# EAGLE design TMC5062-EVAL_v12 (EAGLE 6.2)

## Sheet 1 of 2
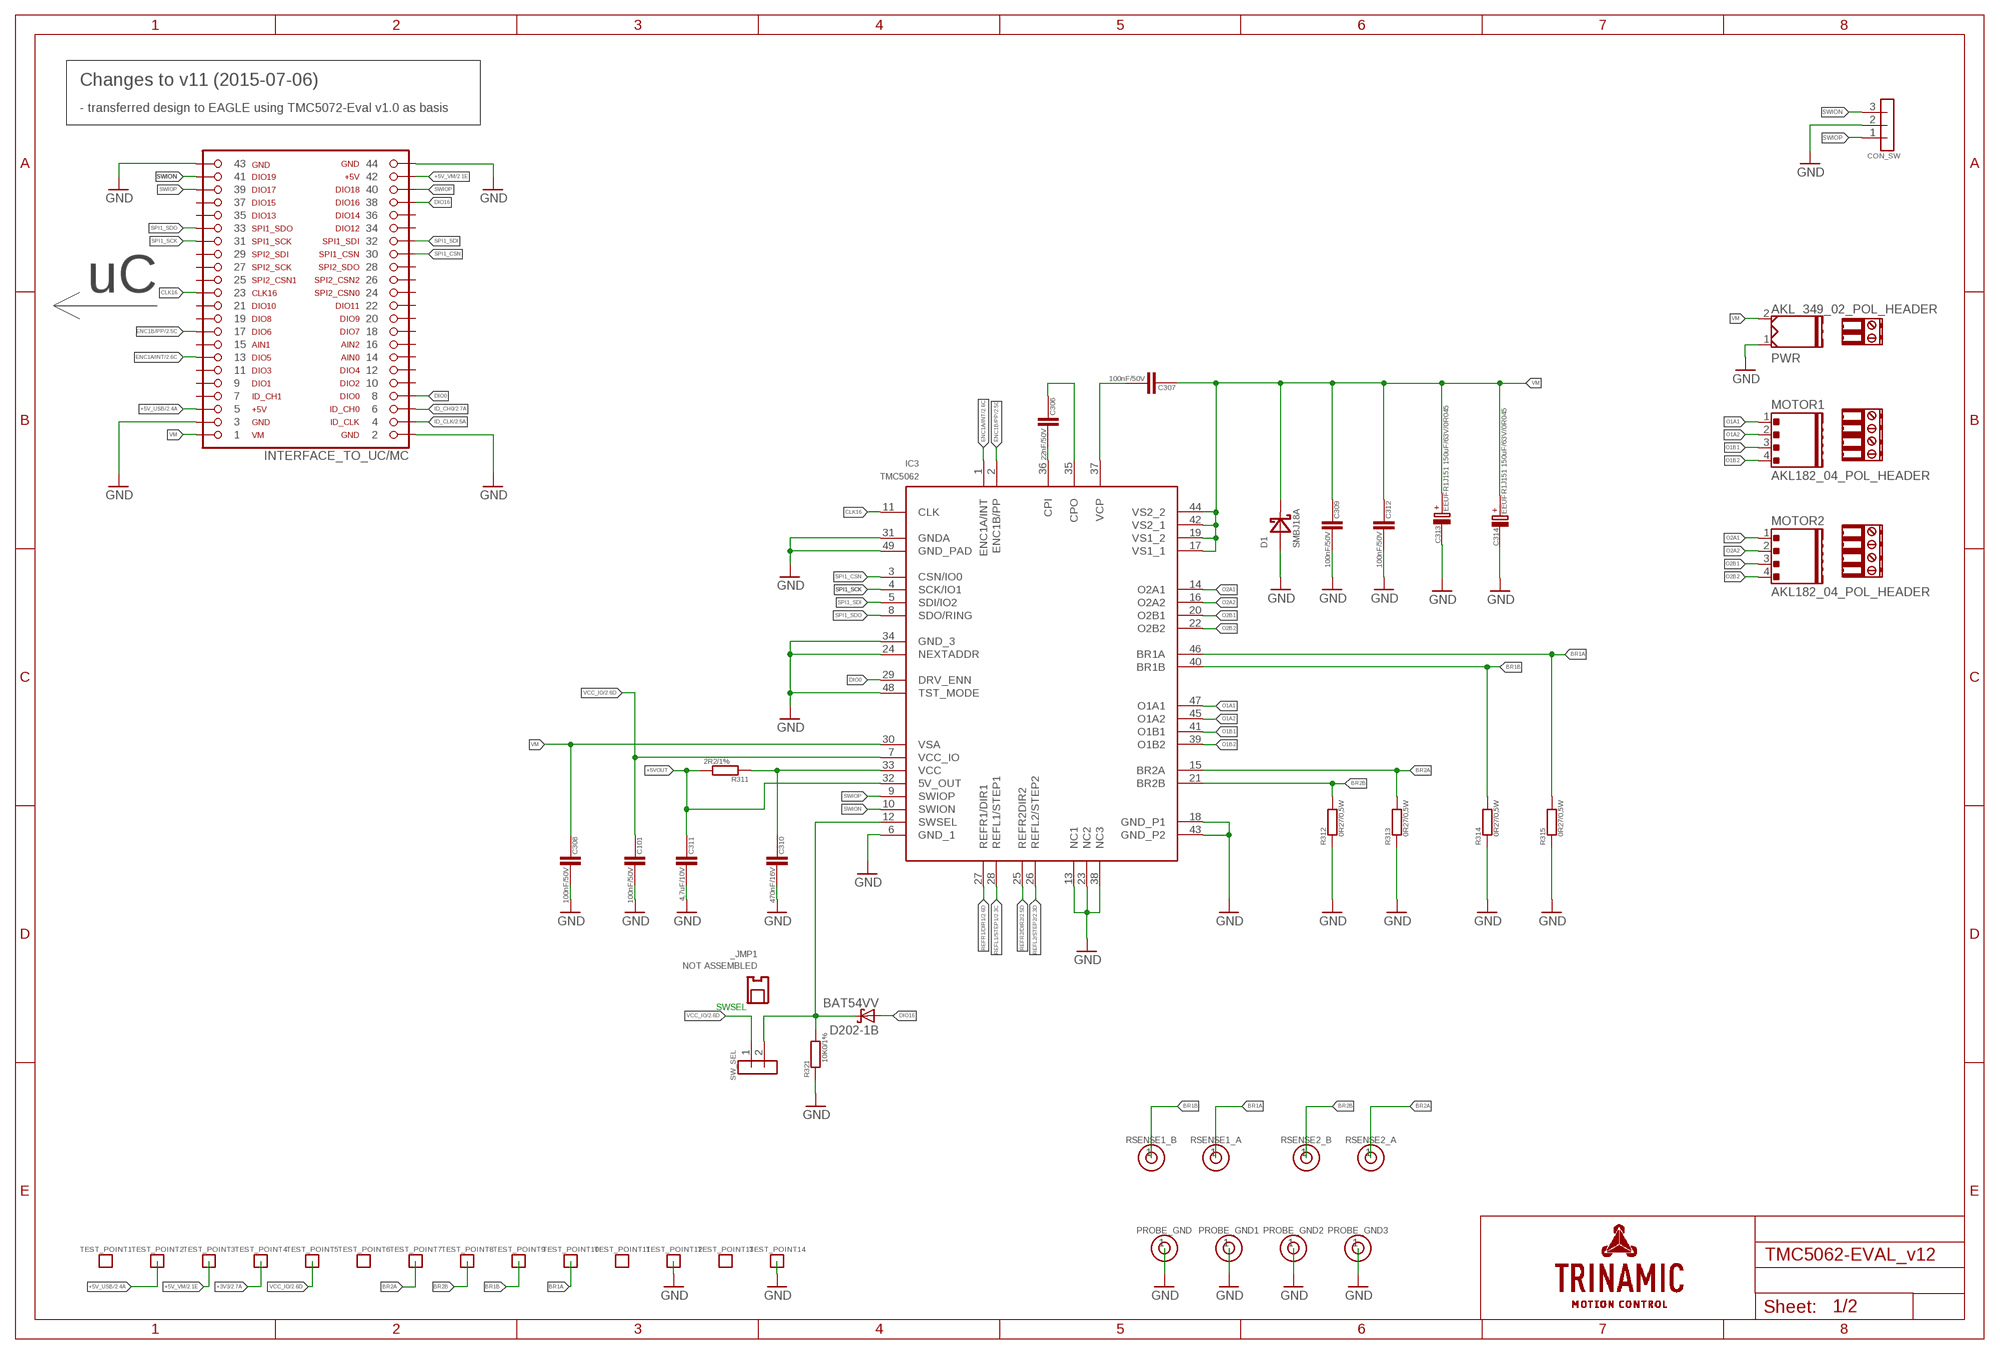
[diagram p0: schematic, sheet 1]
_JMP1 (JUMPER_2.54MM): ADGPN: 3044010200; DATASHEET: http://www.tme.eu/en/Document/d9e6fb6fc4dc34d59ba745016c42e7c7/jumper.pdf; MANUF-CODE-1: JUMPER-B; MANUFACTURER-1: Ninigi; PRICE: 0.11; SUPPLIER: TME; SUPPLIER-CODE: JUMPER-B

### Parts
C101  100nF/50V  C/0603  [0603]
C306  22nF/50V  C/0603  [0603]
C307  100nF/50V  C/0603  [0603]
C308  100nF/50V  C/0603  [0603]
C309  100nF/50V  C/0603  [0603]
C310  470nF/16V  C/0603  [0603]
C311  4,7uF/10V  C/0603  [0603]
C312  100nF/50V  C/0603  [0603]
C313  EEUFR1J151 150uF/63V/0R045  C_POL5X10X12.5  [C_POL_RAD_THT_5X10]
C314  EEUFR1J151 150uF/63V/0R045  C_POL5X10X12.5  [C_POL_RAD_THT_5X10]
CON_SW  NOT ASSEMBLED  3PIN_1ROWNO_FRAME  [3PIN_1ROW_2.54_THT_NO_FRAME]
D1  SMBJ18A  SMBJ  [SMB]
D202-1  BAT54VV  BAS70VV  [SOT666]
IC3  TMC5062  [QFN48]
INTERFACE_TO_UC/MC  FEMALE_HEADER_SMD_2.54_44_PINSHORTPADS_HOLES  [FEMALE_HEADER_SMD_254_44_PIN_SHORTPADS_HOLES]
MOTOR1  AKL182_04_POL_HEADER  [AKL169_04_POL]
MOTOR2  AKL182_04_POL_HEADER  [AKL169_04_POL]
PROBE_GND  NOT ASSEMBLED  1PIN_1ROW  [1PIN_1ROW_THT]
PROBE_GND1  NOT ASSEMBLED  1PIN_1ROW  [1PIN_1ROW_THT]
PROBE_GND2  NOT ASSEMBLED  1PIN_1ROW  [1PIN_1ROW_THT]
PROBE_GND3  NOT ASSEMBLED  1PIN_1ROW  [1PIN_1ROW_THT]
PWR  AKL_349_02_POL_HEADER  [AKL349_02_POL]
R311  2R2/1%  R/0603  [0603]
R312  0R27/0,5W  R  [1206]
R313  0R27/0,5W  R  [1206]
R314  0R27/0,5W  R  [1206]
R315  0R27/0,5W  R  [1206]
R321  10K0/1%  R/0603  [0603]
RSENSE1_A  NOT ASSEMBLED  1PIN_1ROW  [1PIN_1ROW_THT]
RSENSE1_B  NOT ASSEMBLED  1PIN_1ROW  [1PIN_1ROW_THT]
RSENSE2_A  NOT ASSEMBLED  1PIN_1ROW  [1PIN_1ROW_THT]
RSENSE2_B  NOT ASSEMBLED  1PIN_1ROW  [1PIN_1ROW_THT]
SW_SEL  NOT ASSEMBLED  2PIN_1ROWNO_FRAME  [2PIN_1ROW_2.54_THT_NO_FRAME]
TERM1  AKL_330_2_POL_TERMINAL  [EXTRA_TERMINAL]
TERM2  AKL182_04_POL_TERMINAL  [EXTRA_TERMINAL]
TERM3  AKL182_04_POL_TERMINAL  [EXTRA_TERMINAL]
TEST_POINT1  NOT ASSEMBLED  PAD_ROUND  [PAD_R1.2]
TEST_POINT2  NOT ASSEMBLED  PAD_ROUND  [PAD_R1.2]
TEST_POINT3  NOT ASSEMBLED  PAD_ROUND  [PAD_R1.2]
TEST_POINT4  NOT ASSEMBLED  PAD_ROUND  [PAD_R1.2]
TEST_POINT5  NOT ASSEMBLED  PAD_ROUND  [PAD_R1.2]
TEST_POINT6  NOT ASSEMBLED  PAD_ROUND  [PAD_R1.2]
TEST_POINT7  NOT ASSEMBLED  PAD_ROUND  [PAD_R1.2]
TEST_POINT8  NOT ASSEMBLED  PAD_ROUND  [PAD_R1.2]
TEST_POINT9  NOT ASSEMBLED  PAD_ROUND  [PAD_R1.2]
TEST_POINT10  NOT ASSEMBLED  PAD_ROUND  [PAD_R1.2]
TEST_POINT11  NOT ASSEMBLED  PAD_ROUND  [PAD_R1.2]
TEST_POINT12  NOT ASSEMBLED  PAD_ROUND  [PAD_R1.2]
TEST_POINT13  NOT ASSEMBLED  PAD_ROUND  [PAD_R1.2]
TEST_POINT14  NOT ASSEMBLED  PAD_ROUND  [PAD_R1.2]

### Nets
+3V3: TEST_POINT4.P$1 ; also sheet 2
+5V_USB: INTERFACE_TO_UC/MC.5 TEST_POINT2.P$1 ; also sheet 2
+5V_VM: INTERFACE_TO_UC/MC.42 TEST_POINT3.P$1 ; also sheet 2
+5VOUT: C311.2 IC3.32(5V_OUT) R311.2
BR1A: IC3.46(BR1A) R315.2 RSENSE1_A.1 TEST_POINT10.P$1
BR1B: IC3.40(BR1B) R314.2 RSENSE1_B.1 TEST_POINT9.P$1
BR2A: IC3.15(BR2A) R313.2 RSENSE2_A.1 TEST_POINT7.P$1
BR2B: IC3.21(BR2B) R312.2 RSENSE2_B.1 TEST_POINT8.P$1
CLK16: IC3.11(CLK) INTERFACE_TO_UC/MC.23
CPI: C306.1 IC3.36(CPI)
CPO: C306.2 IC3.35(CPO)
DIO0: IC3.29(DRV_ENN) INTERFACE_TO_UC/MC.8
DIO16: D202-1.2(B:A) INTERFACE_TO_UC/MC.38
ENC1A/INT: IC3.1(ENC1A/INT) INTERFACE_TO_UC/MC.13 ; also sheet 2
ENC1B/PP: IC3.2(ENC1B/PP) INTERFACE_TO_UC/MC.17 ; also sheet 2
GND: C101.1 C308.1 C309.1 C310.1 C311.1 C312.1 C313.- C314.- CON_SW.2 D1.A IC3.6(GND_1) IC3.13(NC1) IC3.18(GND_P1) IC3.23(NC2) IC3.24(NEXTADDR) IC3.31(GNDA) IC3.34(GND_3) IC3.38(NC3) IC3.43(GND_P2) IC3.48(TST_MODE) IC3.49(GND_PAD) INTERFACE_TO_UC/MC.2 INTERFACE_TO_UC/MC.3 INTERFACE_TO_UC/MC.43 INTERFACE_TO_UC/MC.44 PROBE_GND1.1 PROBE_GND2.1 PROBE_GND3.1 PROBE_GND.1 PWR.1 R312.1 R313.1 R314.1 R315.1 R321.1 TEST_POINT12.P$1 TEST_POINT14.P$1 ; also sheet 2
ID_CH0: INTERFACE_TO_UC/MC.6 ; also sheet 2
ID_CLK: INTERFACE_TO_UC/MC.4 ; also sheet 2
O1A1: IC3.47(O1A1) MOTOR1.1
O1A2: IC3.45(O1A2) MOTOR1.2
O1B1: IC3.41(O1B1) MOTOR1.3
O1B2: IC3.39(O1B2) MOTOR1.4
O2A1: IC3.14(O2A1) MOTOR2.1
O2A2: IC3.16(O2A2) MOTOR2.2
O2B1: IC3.20(O2B1) MOTOR2.3
O2B2: IC3.22(O2B2) MOTOR2.4
REFL1/STEP1: IC3.28(REFL1/STEP1) ; also sheet 2
REFL2/STEP2: IC3.26(REFL2/STEP2) ; also sheet 2
REFR1/DIR1: IC3.27(REFR1/DIR1) ; also sheet 2
REFR2/DIR2: IC3.25(REFR2DIR2) ; also sheet 2
SPI1_CSN: IC3.3(CSN/IO0) INTERFACE_TO_UC/MC.30
SPI1_SCK: IC3.4(SCK/IO1) INTERFACE_TO_UC/MC.31
SPI1_SDI: IC3.5(SDI/IO2) INTERFACE_TO_UC/MC.32
SPI1_SDO: IC3.8(SDO/RING) INTERFACE_TO_UC/MC.33
SWION: CON_SW.3 IC3.10(SWION) INTERFACE_TO_UC/MC.41
SWIOP: CON_SW.1 IC3.9(SWIOP) INTERFACE_TO_UC/MC.39 INTERFACE_TO_UC/MC.40
SWSEL: D202-1.5(B:C) IC3.12(SWSEL) R321.2 SW_SEL.2
VCC: C310.2 IC3.33(VCC) R311.1
VCC_IO: C101.2 IC3.7(VCC_IO) SW_SEL.1 TEST_POINT5.P$1 ; also sheet 2
VCP: C307.1 IC3.37(VCP)
VM: C307.2 C308.2 C309.2 C312.2 C313.+ C314.+ D1.C IC3.17(VS1_1) IC3.19(VS1_2) IC3.30(VSA) IC3.42(VS2_1) IC3.44(VS2_2) INTERFACE_TO_UC/MC.1 PWR.2
Unconnected: D202-1.1(A:A) D202-1.3(C:A) D202-1.4(C:C) D202-1.6(A:C) INTERFACE_TO_UC/MC.7 INTERFACE_TO_UC/MC.9 INTERFACE_TO_UC/MC.10 INTERFACE_TO_UC/MC.11 INTERFACE_TO_UC/MC.12 INTERFACE_TO_UC/MC.14 INTERFACE_TO_UC/MC.15 INTERFACE_TO_UC/MC.16 INTERFACE_TO_UC/MC.18 INTERFACE_TO_UC/MC.19 INTERFACE_TO_UC/MC.20 INTERFACE_TO_UC/MC.21 INTERFACE_TO_UC/MC.22 INTERFACE_TO_UC/MC.24 INTERFACE_TO_UC/MC.25 INTERFACE_TO_UC/MC.26 INTERFACE_TO_UC/MC.27 INTERFACE_TO_UC/MC.28 INTERFACE_TO_UC/MC.29 INTERFACE_TO_UC/MC.34 INTERFACE_TO_UC/MC.35 INTERFACE_TO_UC/MC.36 INTERFACE_TO_UC/MC.37 TEST_POINT1.P$1 TEST_POINT6.P$1 TEST_POINT11.P$1 TEST_POINT13.P$1

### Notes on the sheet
- Changes to v11 (2015-07-06)
- - transferred design to EAGLE using TMC5072-Eval v1.0 as basis
- uC
- SWSEL

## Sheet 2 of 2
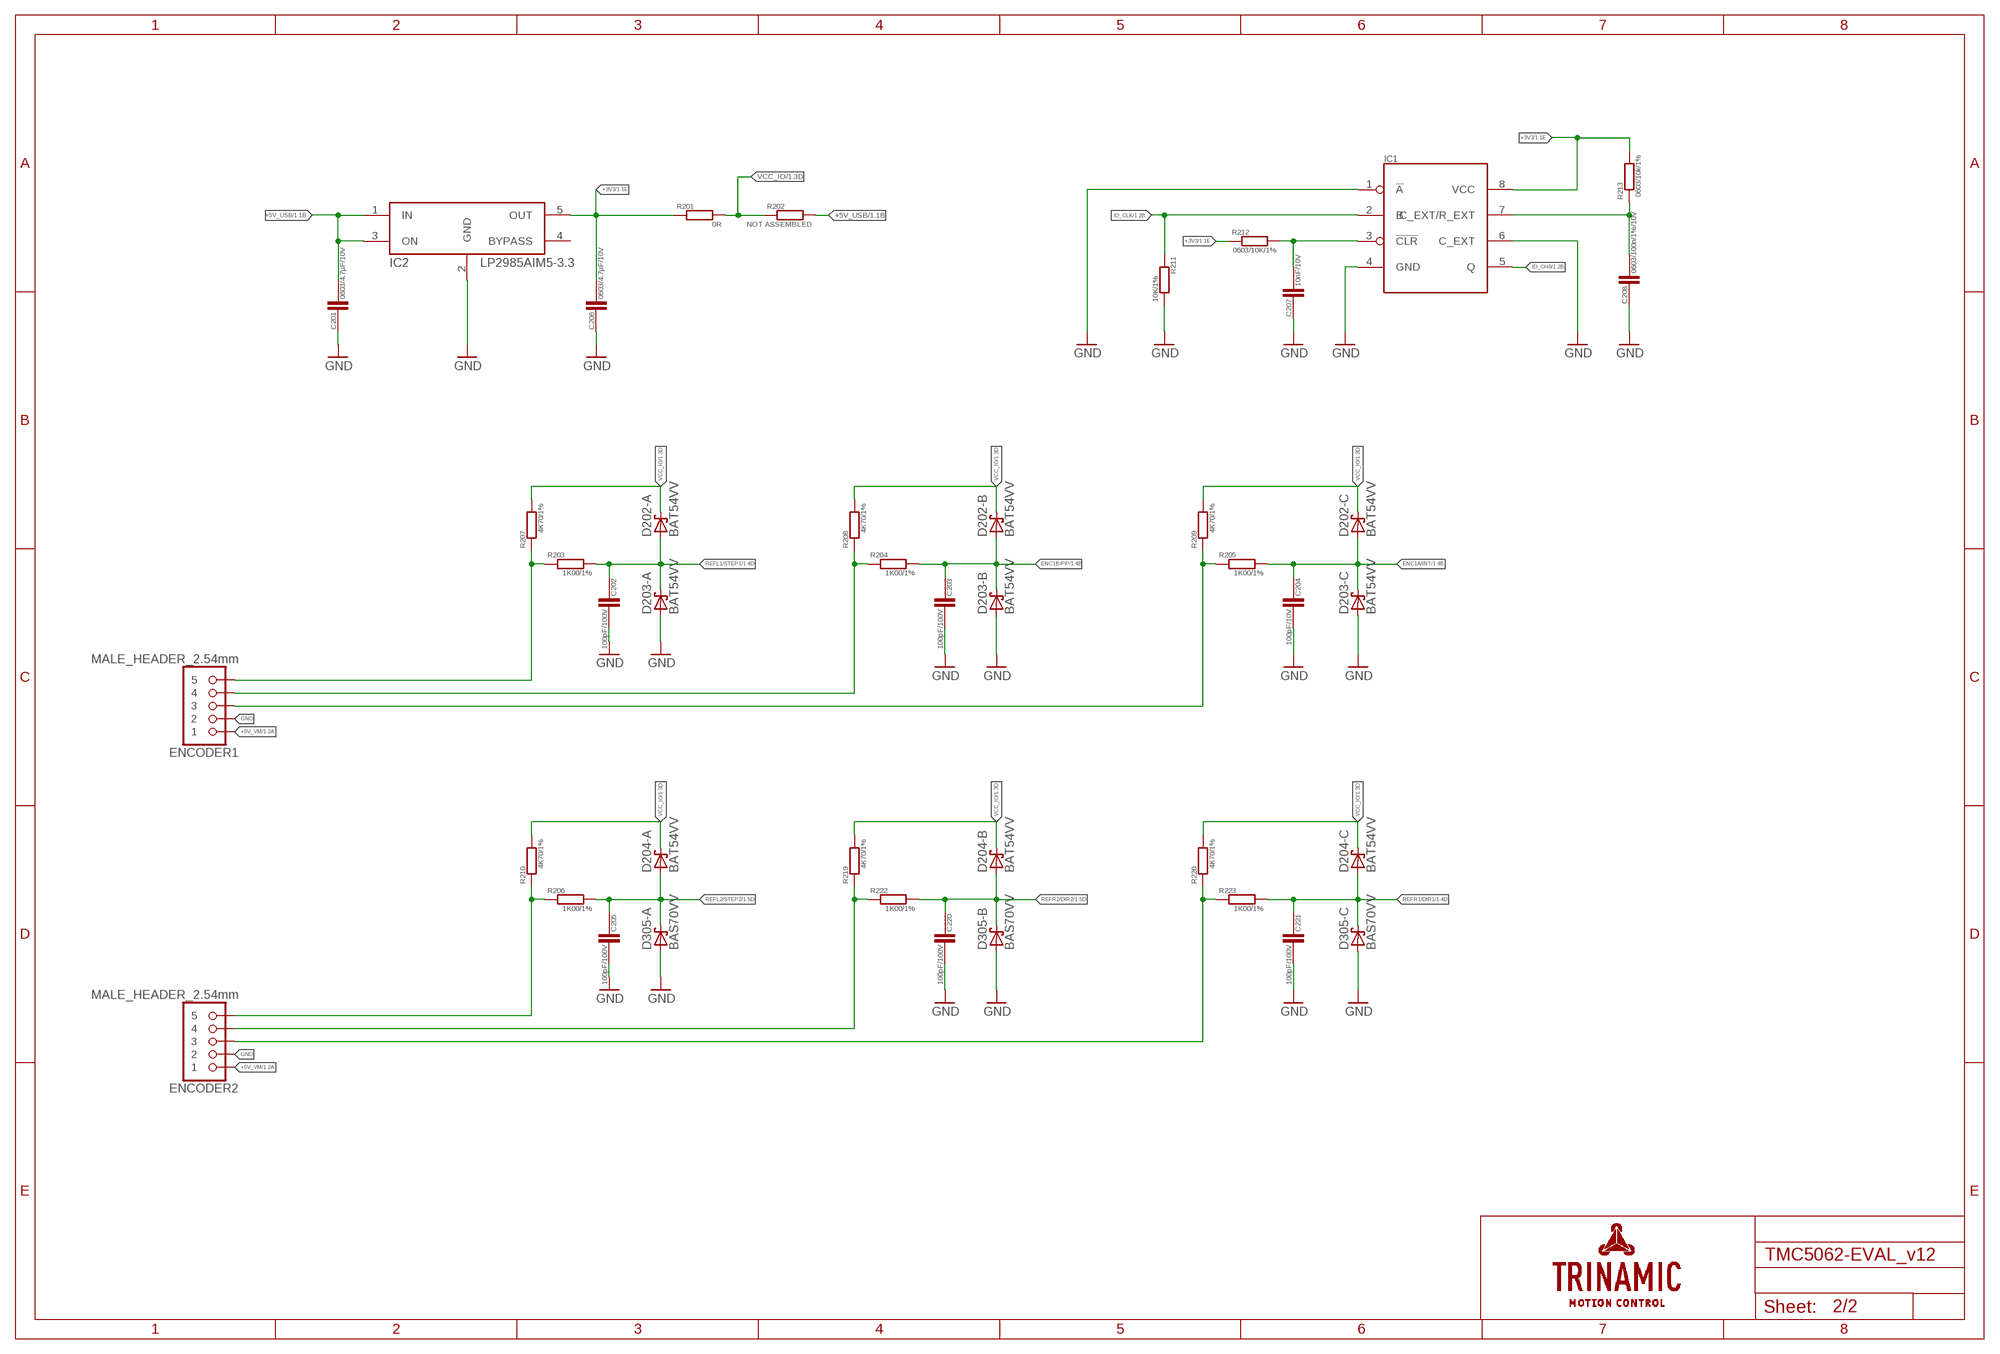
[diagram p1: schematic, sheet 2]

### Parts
C201  0603/4.7µF/10V  RCL_C/0603  [RCL_0603]
C202  100pF/100V  C/0603  [0603]
C203  100pF/100V  C/0603  [0603]
C204  100pF/10V  C/0603  [0603]
C205  100pF/100V  C/0603  [0603]
C206  0603/4.7µF/10V  RCL_C/0603  [RCL_0603]
C207  10nF/10V  RCL_C/0603  [RCL_0603]
C208  0603/100n/1%/10V  RCL_C/0603  [RCL_0603]
C220  100pF/100V  C/0603  [0603]
C221  100pF/100V  C/0603  [0603]
D202-  BAT54VV  BAS70VV  [SOT666]
D203-  BAT54VV  BAS70VV  [SOT666]
D204-  BAT54VV  BAS70VV  [SOT666]
D305-  BAS70VV  [SOT666]
ENCODER1  MALE_HEADER_2.54mm  5PIN_1ROWTHT  [5PIN_1ROW_2.54_THT]
ENCODER2  MALE_HEADER_2.54mm  5PIN_1ROWTHT  [5PIN_1ROW_2.54_THT]
IC1  SN74LVC1G123DCTR  [SN74LVC1G123DCTR]
IC2  LP2985AIM5-3.3  [SOT23-5]
R201  0R  R/0603  [0603]
R202  NOT ASSEMBLED  R/0603  [0603]
R203  1K00/1%  R/0603  [0603]
R204  1K00/1%  R/0603  [0603]
R205  1K00/1%  R/0603  [0603]
R206  1K00/1%  R/0603  [0603]
R207  4K70/1%  R/0603  [0603]
R208  4K70/1%  R/0603  [0603]
R209  4K70/1%  R/0603  [0603]
R210  4K70/1%  R/0603  [0603]
R211  10K/1%  RCL_R/0603  [RCL_0603]
R212  0603/10K/1%  RCL_R/0603  [RCL_0603]
R213  0603/10k/1%  RCL_R/0603  [RCL_0603]
R219  4K70/1%  R/0603  [0603]
R220  4K70/1%  R/0603  [0603]
R222  1K00/1%  R/0603  [0603]
R223  1K00/1%  R/0603  [0603]

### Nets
+3V3: C206.1 IC1.8(VCC) IC2.5(OUT) R201.1 R212.1 R213.2 ; also sheet 1
+5V_USB: C201.1 IC2.1(IN) IC2.3(ON) R202.2 ; also sheet 1
+5V_VM: ENCODER1.1 ENCODER2.1 ; also sheet 1
ENC1A/INT: C204.2 D202-.3(C:A) D203-.4(C:C) R205.2 ; also sheet 1
ENC1B/PP: C203.2 D202-.2(B:A) D203-.5(B:C) R204.2 ; also sheet 1
GND: C201.2 C202.1 C203.1 C204.1 C205.1 C206.2 C207.2 C208.2 C220.1 C221.1 D203-.1(A:A) D203-.2(B:A) D203-.3(C:A) D305-.1(A:A) D305-.2(B:A) D305-.3(C:A) ENCODER1.2 ENCODER2.2 IC1.1(!A) IC1.4(GND) IC1.6(C_EXT) IC2.2(GND) R211.2 ; also sheet 1
ID_CH0: IC1.5(Q) ; also sheet 1
ID_CLK: IC1.2(B) R211.1 ; also sheet 1
N$1: C207.1 IC1.3(!CLR) R212.2
N$2: C208.1 IC1.7(C_EXT/R_EXT) R213.1
N$3: ENCODER1.5 R203.1 R207.1
N$4: ENCODER1.4 R204.1 R208.1
N$5: ENCODER1.3 R205.1 R209.1
N$6: ENCODER2.5 R206.1 R210.1
N$7: ENCODER2.4 R219.1 R222.1
N$8: ENCODER2.3 R220.1 R223.1
REFL1/STEP1: C202.2 D202-.1(A:A) D203-.6(A:C) R203.2 ; also sheet 1
REFL2/STEP2: C205.2 D204-.1(A:A) D305-.6(A:C) R206.2 ; also sheet 1
REFR1/DIR1: C221.2 D204-.3(C:A) D305-.4(C:C) R223.2 ; also sheet 1
REFR2/DIR2: C220.2 D204-.2(B:A) D305-.5(B:C) R222.2 ; also sheet 1
VCC_IO: D202-.4(C:C) D202-.5(B:C) D202-.6(A:C) D204-.4(C:C) D204-.5(B:C) D204-.6(A:C) R201.2 R202.1 R207.2 R208.2 R209.2 R210.2 R219.2 R220.2 ; also sheet 1
Unconnected: IC2.4(BYPASS)

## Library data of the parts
C101 C202-C205 C220 C221 C306-C312 = _TMC_TE_RCL:C
C201 C206-C208 = TMC_EVAL_driver_TE_v01:RCL_C
C313 C314 = _TMC_TE_RCL:C_POL
CON_SW = _TMC_TE_con:3PIN_1ROW
D1 = _TMC_TE_D:SMBJ
D202- D202-1 D203- D204- D305- = diode:BAS70VV: Silicon Schottky Diodes General-purpose diode for high-speed switching Source: BAS70_1PS7XSB70_SER_8.pdf
ENCODER1 ENCODER2 = _TMC_TE_con:5PIN_1ROW
IC1 = TMC_EVAL_driver_TE_v01:SN74LVC1G123DCTR
IC2 = TMC_EVAL_driver_TE_v01:LP2985AIM5-3.3
IC3 = trinamic:TMC5062
INTERFACE_TO_UC/MC = _TMC_TE_con:FEMALE_HEADER_SMD_2.54_44_PIN; 1_PARTNUMBER: 098-3-044-1-NFX-YT0; 1_SUPPLIER: MPE Garry; 2_PARTNUMBER: HLE-122-02-F-DV-A; 2_SUPPLIER: Samtec
MOTOR1 MOTOR2 = _TMC_TE_con:AKL182_04_POL_HEADER: AKL header, shrouted, 4 pins; 1_PARTNUMBER: 31182104; 1_SUPPLIER: RIA CONNECT; 2_PARTNUMBER: AKL 182-04; 2_SUPPLIER: Reichelt
PROBE_GND PROBE_GND1-PROBE_GND3 RSENSE1_A RSENSE1_B RSENSE2_A RSENSE2_B = _TMC_TE_con:1PIN_1ROW
PWR = _TMC_TE_con:AKL_349_02_POL_HEADER: AKL header, shrouted, 2 pins; 1_PARTNUMBER: 31330102; 1_SUPPLIER: RIA CONNECT; 2_PARTNUMBER: AKL 330-02; 2_SUPPLIER: REICHELT
R201-R210 R219 R220 R222 R223 R311-R315 R321 = _TMC_TE_RCL:R
R211-R213 = TMC_EVAL_driver_TE_v01:RCL_R
SW_SEL = _TMC_TE_con:2PIN_1ROW
TERM1 = _TMC_TE_con:AKL_330_2_POL_TERMINAL: AKL terminal, 2 pins; 1_PARTNUMBER: 31349102; 1_SUPPLIER: RIA CONNECT; 2_PARTNUMBER: AKL 349-02; 2_SUPPLIER: Reichelt
TERM2 TERM3 = _TMC_TE_con:AKL182_04_POL_TERMINAL: AKL terminal, 4 pins; 1_PARTNUMBER: 31169104; 1_SUPPLIER: RIA CONNECT; 2_PARTNUMBER: AKL 169-04; 2_SUPPLIER: Reichelt
TEST_POINT1-TEST_POINT14 = _TMC_TE_PADS:PAD_ROUND

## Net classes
0 default: width 0.254 mm, drill 0.15 mm

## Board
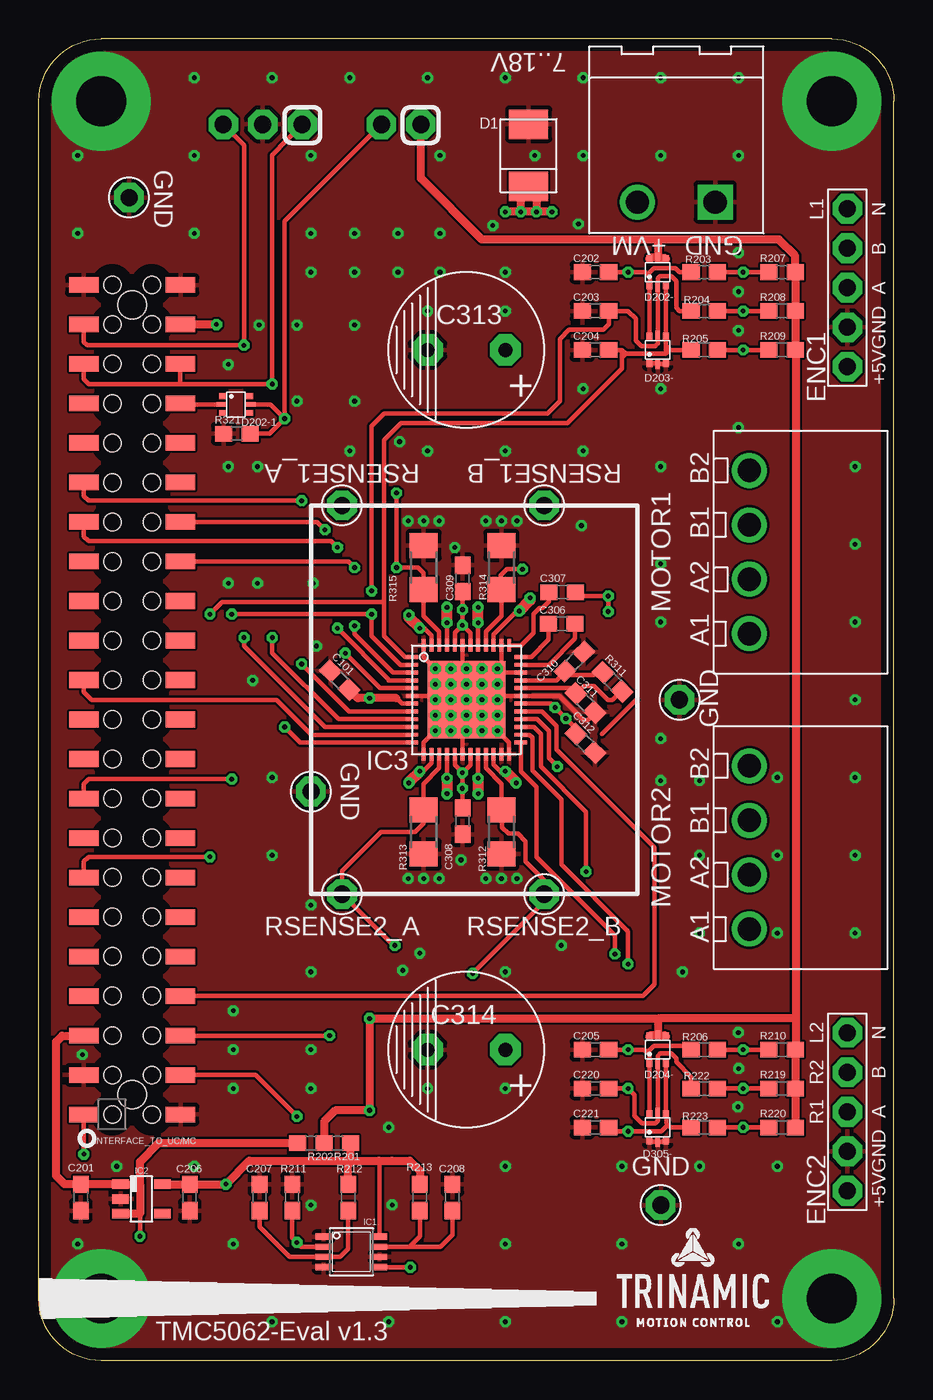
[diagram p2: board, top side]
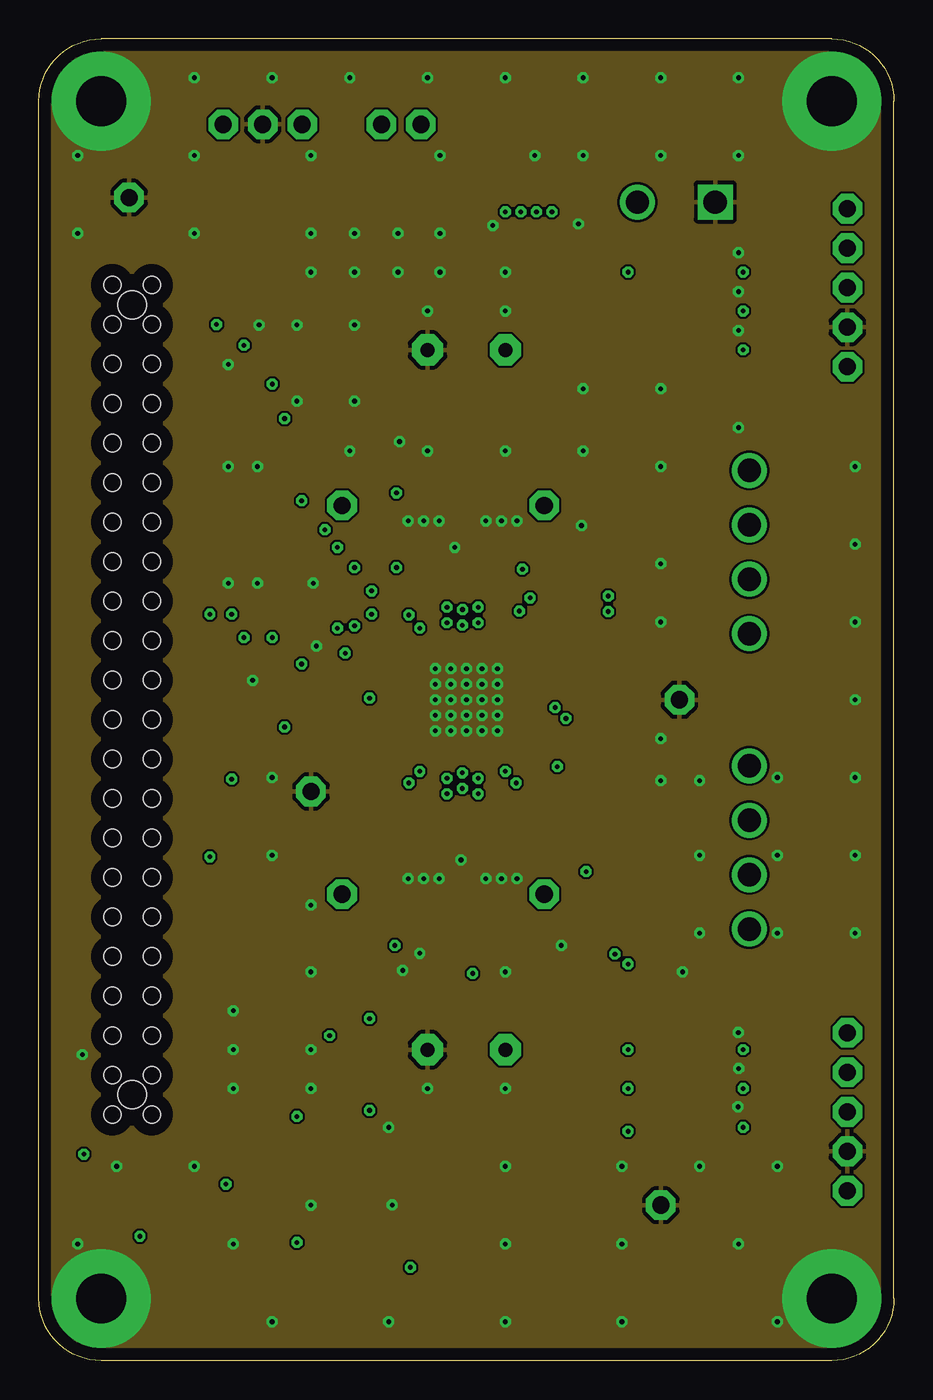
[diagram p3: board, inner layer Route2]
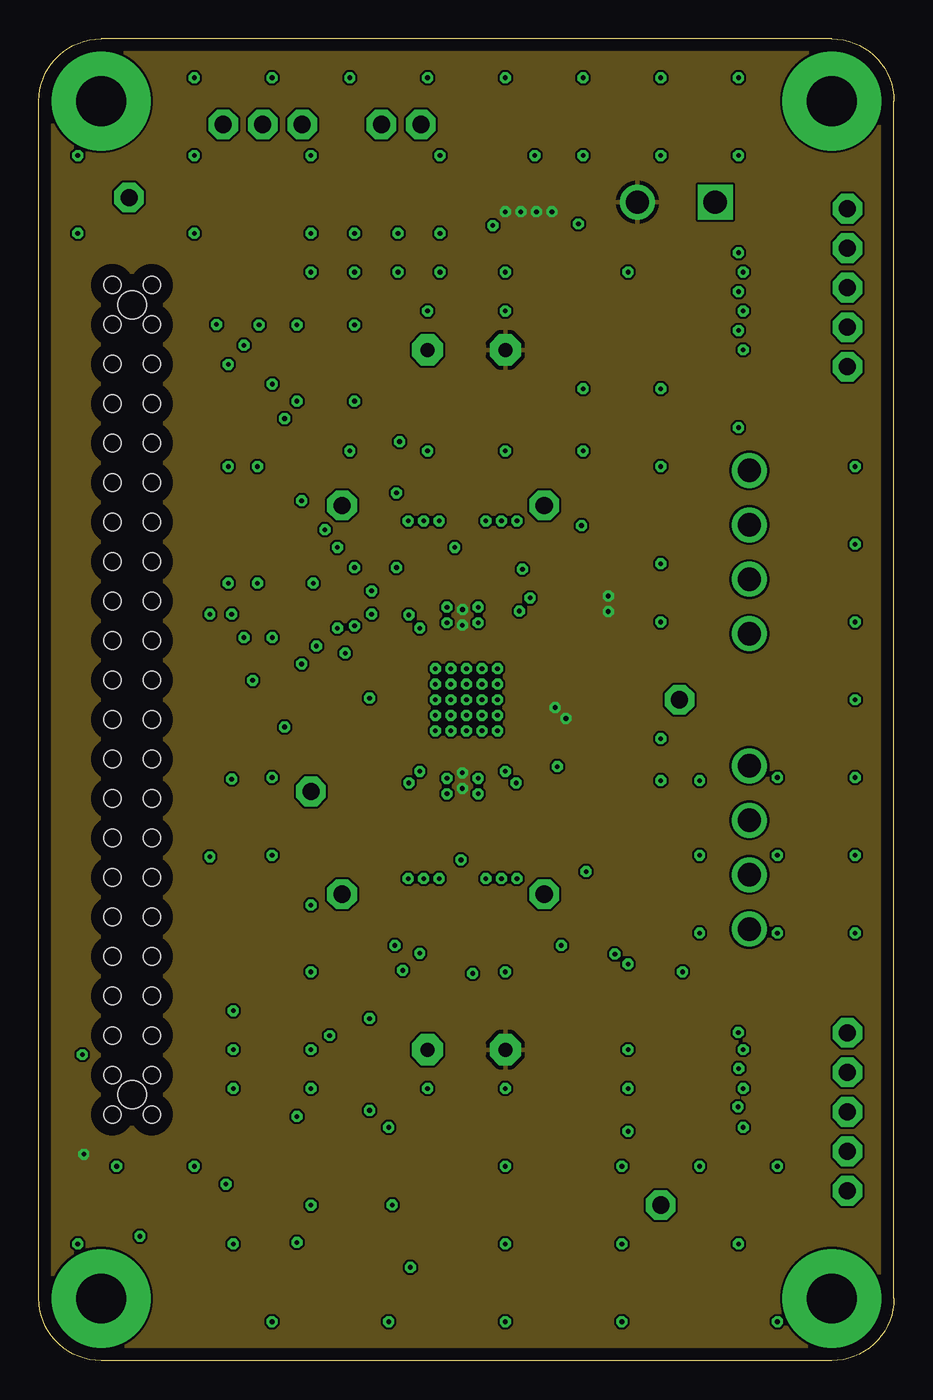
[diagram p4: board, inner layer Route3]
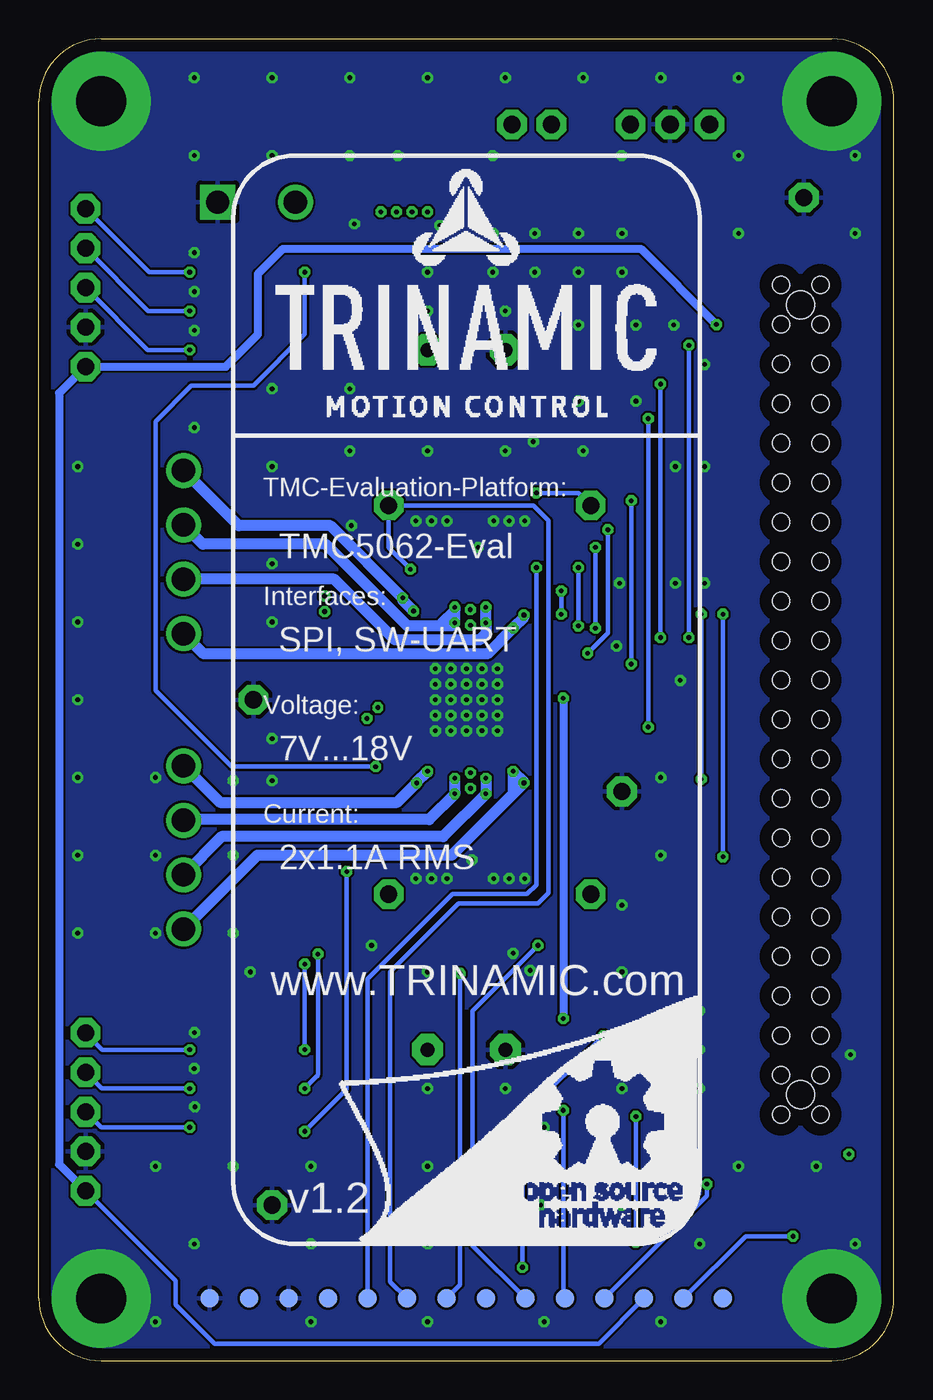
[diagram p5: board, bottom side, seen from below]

Size 55 x 85 mm. Coordinates in mm from the lower left corner, seen from the top.
Outline: 51,0 4,0 arc-90 0,4 0,81 arc-90 4,85 51,85 arc-90 55,81 55,4 arc-90 51,0
Copper layers (1*2*3*16): Top 0.018mm / dielectric 0.36mm / Route2 0.035mm / dielectric 0.71mm / Route3 0.035mm / dielectric 0.2mm / Bottom 0.018mm
Design rules: minimum track width 0.15mm, minimum drill 0.25mm, track to track 0.15mm, track to pad 0.15mm, pad to pad 0.1mm, via to via 0.15mm, smd to smd 0mil, copper to edge 0.8mm, drill to drill 8mil, minimum pad ring 10mil, minimum via ring 8mil, stop-mask expansion 4mil, vias tented up to drill 0.4mm, thermal gap 10mil

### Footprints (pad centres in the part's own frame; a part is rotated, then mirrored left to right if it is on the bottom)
0603 = smd 1.1 x 1: 1 -0.85,0; 2 0.85,0
RCL_0603 = smd 1.1 x 1: 1 -0.85,0; 2 0.85,0
C_POL_RAD_THT_5X10 = drill 0.9 pad 2 octagon: + 2.5,0; - -2.5,0
3PIN_1ROW_2.54_THT_NO_FRAME = drill 1.1 pad 1.9 octagon: 1 -2.54,0; 2 0,0; 3 2.54,0
SMB = smd 1.9 x 2.5: A 2,0; C -2,0
SOT666 = smd 0.375 x 0.5: 1 -0.537,-0.85; 3 0.538,-0.85; 4 0.538,0.849; 6 -0.538,0.85 | smd 0.3 x 0.65: 2 0,-0.923; 5 0,0.925
5PIN_1ROW_2.54_THT = drill 1.1 pad 1.9 octagon: 1 -5.08,0; 2 -2.54,0; 3 0,0; 4 2.54,0; 5 5.08,0
SN74LVC1G123DCTR = smd 0.4 x 1: 1 -0.975,-1.8; 2 -0.325,-1.8; 3 0.325,-1.8; 4 0.975,-1.8; 5 0.975,1.8; 6 0.325,1.8; 7 -0.325,1.8; 8 -0.975,1.8
SOT23-5 = smd 0.6 x 1.05: 1 -0.95,-1.35; 2 0,-1.35; 3 0.95,-1.35; 4 0.95,1.35; 5 -0.95,1.35
QFN48 = smd 0.25 x 0.8: 1 -2.75,-3.5; 2 -2.25,-3.5; 3 -1.75,-3.5; 4 -1.25,-3.5; 5 -0.75,-3.5; 6 -0.25,-3.5; 7 0.25,-3.5; 8 0.75,-3.5; 9 1.25,-3.5; 10 1.75,-3.5; 11 2.25,-3.5; 12 2.75,-3.5; 25 2.75,3.5; 26 2.25,3.5; 27 1.75,3.5; 28 1.25,3.5; 29 0.75,3.5; 30 0.25,3.5; 31 -0.25,3.5; 32 -0.75,3.5; 33 -1.25,3.5; 34 -1.75,3.5; 35 -2.25,3.5; 36 -2.75,3.5 | smd 0.8 x 0.25: 13 3.5,-2.75; 14 3.5,-2.25; 15 3.5,-1.75; 16 3.5,-1.25; 17 3.5,-0.75; 18 3.5,-0.25; 19 3.5,0.25; 20 3.5,0.75; 21 3.5,1.25; 22 3.5,1.75; 23 3.5,2.25; 24 3.5,2.75; 37 -3.5,2.75; 38 -3.5,2.25; 39 -3.5,1.75; 40 -3.5,1.25; 41 -3.5,0.75; 42 -3.5,0.25; 43 -3.5,-0.25; 44 -3.5,-0.75; 45 -3.5,-1.25; 46 -3.5,-1.75; 47 -3.5,-2.25; 48 -3.5,-2.75 | smd 5 x 5: 49 0,0
FEMALE_HEADER_SMD_254_44_PIN_SHORTPADS_HOLES = smd 1 x 1.9: 1 -26.67,3.11; 2 -26.67,-3.11; 3 -24.13,3.11; 4 -24.13,-3.11; 5 -21.59,3.11; 6 -21.59,-3.11; 7 -19.05,3.11; 8 -19.05,-3.11; 9 -16.51,3.11; 10 -16.51,-3.11; 11 -13.97,3.11; 12 -13.97,-3.11; 13 -11.43,3.11; 14 -11.43,-3.11; 15 -8.89,3.11; 16 -8.89,-3.11; 17 -6.35,3.11; 18 -6.35,-3.11; 19 -3.81,3.11; 20 -3.81,-3.11; 21 -1.27,3.11; 22 -1.27,-3.11; 23 1.27,3.11; 24 1.27,-3.11; 25 3.81,3.11; 26 3.81,-3.11; 27 6.35,3.11; 28 6.35,-3.11; 29 8.89,3.11; 30 8.89,-3.11; 31 11.43,3.11; 32 11.43,-3.11; 33 13.97,3.11; 34 13.97,-3.11; 35 16.51,3.11; 36 16.51,-3.11; 37 19.05,3.11; 38 19.05,-3.11; 39 21.59,3.11; 40 21.59,-3.11; 41 24.13,3.11; 42 24.13,-3.11; 43 26.67,3.11; 44 26.67,-3.11 | hole 1.8: -25.4,0; 25.4,0 | hole 1.1: -26.67,1.27; -24.13,1.27; -21.59,1.27; -19.05,1.27; -16.51,1.27; -13.97,1.27; -11.43,1.27; -8.89,1.27; -6.35,1.27; -3.81,1.27; -1.27,1.27; 1.27,1.27; 3.81,1.27; 6.35,1.27; 8.89,1.27; 11.43,1.27; 13.97,1.27; 16.51,1.27; 19.05,1.27; 21.59,1.27; 24.13,1.27; 26.67,1.27; -26.67,-1.27; -24.13,-1.27; -21.59,-1.27; -19.05,-1.27; -16.51,-1.27; -13.97,-1.27; -11.43,-1.27; -8.89,-1.27; -6.35,-1.27; -3.81,-1.27; -1.27,-1.27; 1.27,-1.27; 3.81,-1.27; 6.35,-1.27; 8.89,-1.27; 11.43,-1.27; 13.97,-1.27; 16.51,-1.27; 19.05,-1.27; 21.59,-1.27; 24.13,-1.27; 26.67,-1.27
AKL169_04_POL = drill 1.5: 1 -5.25,3.3; 2 -1.75,3.3; 3 1.75,3.3; 4 5.25,3.3
1PIN_1ROW_THT = drill 1.1 pad 1.9 octagon: 1 0,0
AKL349_02_POL = drill 1.5 square: 1 -2.5,4 | drill 1.5: 2 2.5,4
1206 = smd 1.6 x 1.803: 1 -1.422,0; 2 1.422,0
2PIN_1ROW_2.54_THT_NO_FRAME = drill 1.1 pad 1.9 octagon: 1 -1.27,0; 2 1.27,0
PAD_R1.2 = smd 1.2 x 1.2: P$1 0,0

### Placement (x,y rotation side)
C101  19.35,43.76 315 top
C201  2.7,10.5 270 top
C202  35.8,70 0 top
C203  35.8,67.5 0 top
C204  35.8,65 0 top
C205  35.8,20 0 top
C206  9.7,10.5 270 top
C207  14.2,10.5 90 top
C208  26.6,10.5 90 top
C220  35.8,17.5 0 top
C221  35.8,15 0 top
C306  33.63,47.38 0 top
C307  33.66,49.42 0 top
C308  27.25,34.7 90 top
C309  27.25,50.3 270 top
C310  34.44,44.96 225 top
C311  35.15,42.3 135 top
C312  35.15,39.7 135 top
C313  27.5,65 0 top
C314  27.5,20 0 top
CON_SW  14.4,79.5 180 top
D1  31.5,77.5 90 top
D202-  39.8,70 0 top
D202-1  12.68,61.49 270 top
D203-  39.8,65 0 top
D204-  39.8,20 0 top
D305-  39.8,15 0 top
ENCODER1  52,69 90 top
ENCODER2  52,16 90 top
IC1  20.1,7 270 top
IC2  6.6,10.4 270 top
IC3  27.5,42.5 270 top
INTERFACE_TO_UC/MC  6,42.5 90 top
MOTOR1  49,52 90 top
MOTOR2  49,33 90 top
PROBE_GND  41.2,42.5 0 top
PROBE_GND1  17.5,36.6 180 top
PROBE_GND2  5.8,74.8 270 top
PROBE_GND3  40,10 0 top
PWR  41,78.5 180 top
R201  19.2,14 180 top
R202  17.5,14 180 top
R203  42.8,70 180 top
R204  42.8,67.5 180 top
R205  42.8,65 180 top
R206  42.8,20 180 top
R207  47.8,70 0 top
R208  47.8,67.5 0 top
R209  47.8,65 0 top
R210  47.8,20 0 top
R211  16.3,10.5 90 top
R212  19.9,10.5 270 top
R213  24.5,10.5 90 top
R219  47.8,17.5 0 top
R220  47.8,15 0 top
R222  42.8,17.5 180 top
R223  42.8,15 180 top
R311  36.9,43.65 315 top
R312  29.75,34 90 top
R313  24.75,34 90 top
R314  29.75,51 270 top
R315  24.75,51 270 top
R321  12.74,59.61 0 top
RSENSE1_A  19.5,55 0 top
RSENSE1_B  32.5,55 0 top
RSENSE2_A  19.5,30 0 top
RSENSE2_B  32.5,30 0 top
SW_SEL  23.3,79.5 180 top
TERM1  0,-2.5 0 top
TERM2  not placed on the board
TERM3  not placed on the board
TEST_POINT1  11,4 0 bottom
TEST_POINT2  13.54,4 0 bottom
TEST_POINT3  16.08,4 0 bottom
TEST_POINT4  18.62,4 0 bottom
TEST_POINT5  21.16,4 0 bottom
TEST_POINT6  26.24,4 0 bottom
TEST_POINT7  23.7,4 0 bottom
TEST_POINT8  28.78,4 0 bottom
TEST_POINT9  31.32,4 0 bottom
TEST_POINT10  33.86,4 0 bottom
TEST_POINT11  36.4,4 0 bottom
TEST_POINT12  38.94,4 0 bottom
TEST_POINT13  41.48,4 0 bottom
TEST_POINT14  44.02,4 0 bottom
U$1  [TMC_EVAL_RIGHT_BAR]  0,0 0 top
U$3  [TMC_EVAL_BACK_NO_DOCU]  55,0 0 bottom

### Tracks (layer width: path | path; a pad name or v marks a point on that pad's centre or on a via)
+3V3  (via drill 0.3 pad 0.3)
  Top 0.3: 23,12.85 22.7,12.85 | IC1.8 21.9,12.81 21.86,12.85
  Top 0.5: IC2.5 C206.1 v12.03,11.35 13.53,12.85 19.9,12.85 | 19.9,12.85 21.86,12.85 22.7,12.85 23.85,12.85 24.5,12.2 R213.2 | R212.1 19.9,12.85 | 19.9,12.85 20.05,13 R201.1
  Bottom 0.3: v12.03,11.35 12.03,10.59 TEST_POINT4.P$1
+5V_USB  (via drill 0.3 pad 0.3)
  Top 0.3: 6.5,9.45 v6.5,8
  Top 0.5: 2.51,20.91 INTERFACE_TO_UC/MC.5 1.5,20.9 1.1,20.5 1.1,11.9 1.65,11.35 C201.1 IC2.1 6.5,11.35 | 6.5,11.35 6.5,9.45 IC2.3 | 6.5,11.35 6.5,12.8 7.7,14 R202.2
  Bottom 0.3: v6.5,8 9.54,8 TEST_POINT2.P$1
+5V_VM  (via drill 0.3 pad 0.3)
  Top 0.5: v11.42,66.63 INTERFACE_TO_UC/MC.42
  Bottom 0.3: TEST_POINT3.P$1 18.98,1.1 43.7,1.1 46.2,3.6 46.2,5.12 ENCODER2.1
  Bottom 0.5: ENCODER2.1 53.7,12.62 53.7,62.22 ENCODER1.1 42.98,63.92 40.9,66 40.9,69.9 39.3,71.5 16.29,71.5 v11.42,66.63
+5VOUT
  Top 0.3: IC3.32 34.2,43.25 C311.2 35.05,43.4 35.7,43.4 36.6,42.5 36.9,42.5 37.45,43.05 R311.2
BR1A  (via drill 0.3, 0.3 pad 0.3)
  Top 0.3: IC3.46 25.75,46.9 24.75,47.9 R315.2 24.75,50.65 24.4,51 v23,51 v23,55.8
  Bottom 0.3: v23,51 23,30.6 23.6,30 28.4,30 33.86,24.54 TEST_POINT10.P$1 33.8,4.06 | v23,55.8 20.41,55.8 arc45 20.23,55.73 RSENSE1_A.1
BR1B  (via drill 0.3)
  Top 0.3: IC3.40 28.75,46.9 29.75,47.9 R314.2 29.32,49.58 29.32,49.78 29.58,49.78 29.7,49.9 29.7,50.5 30.1,50.9 v31.1,50.9
  Bottom 0.3: TEST_POINT9.P$1 32.4,5.08 32.4,25.01 28,29.41 22.9,29.41 22.22,30.09 22.22,54.02 23.2,55 RSENSE1_B.1 32.5,52.3 v31.1,50.9
BR2A  (via drill 0.3)
  Top 0.3: IC3.15 25.75,38.1 24.75,37.1 R313.2 24.75,34.55 24.2,34 22,34 19.5,31.5 RSENSE2_A.1 22.8,26.7 v22.9,26.7
  Bottom 0.3: TEST_POINT7.P$1 27.1,7.4 27.1,22.5 v22.9,26.7
BR2B  (via drill 0.3 pad 0.25)
  Top 0.3: IC3.21 28.75,38.1 29.75,37.1 R312.2 29.75,35.25 29.8,35.2 29.8,34.3 30.2,33.9 30.8,33.9 31.3,33.4 31.3,32.1 32.5,30.9 RSENSE2_B.1 32.5,29.61 arc-45 32.43,29.43 v27.9,24.9
  Bottom 0.3: 28.8,4.02 TEST_POINT8.P$1 27.9,4.88 v27.9,24.9
CLK16
  Top 0.3: IC3.11 17.55,40.25 15.3,42.5 3.4,42.5 2.89,43.01 INTERFACE_TO_UC/MC.23
CPI
  Top 0.3: IC3.36 31.67,45.25 32.78,46.37 C306.1
CPO
  Top 0.3: IC3.35 32.81,44.75 34.48,46.42 C306.2
DIO0
  Top 0.3: IC3.29 32.35,41.75 33.3,40.8 33.3,39.3 39.6,33 39.6,24.2 38.85,23.45 INTERFACE_TO_UC/MC.8
DIO16
  Top 0.3: 9.16,61.5 INTERFACE_TO_UC/MC.38 9.17,61.49 D202-1.2
ENC1A/INT  (via drill 0.3 pad 0.3)
  Top 0.3: IC3.1 23.55,45.25 22.2,46.6 22.2,48.8 | INTERFACE_TO_UC/MC.13 2.89,32.09 3.2,32.4 v11,32.4 | D202-.3 D203-.4 40.34,65.28 | C204.2 36.6,65 36.9,64.7 | 40.34,65.28 40.34,64.75 | 36.9,64.75 C204.2 | 22.2,48.8 22.2,59.2 23.3,60.3 34,60.3 37.5,63.8 37.5,64 37.5,64.5 | 22.2,48.8 11.8,48.8 v11,48 | 40.34,64.75 40.59,65 40.62,65 | 40.62,65 R205.2 | 40.34,65.28 40.62,65 | 37.5,65 C204.2 | 37.5,64.5 37.5,65 | 37.5,65 37.75,64.75 | 37.75,64.75 40.34,64.75 | 37.75,64.75 37.5,64.5
  Bottom 0.3: v11,48 v11,32.4
ENC1B/PP  (via drill 0.3, 0.3 pad 0.3)
  Top 0.3: IC3.2 23.25,44.75 21.4,46.6 v21.4,48 v12.4,48 | 41.6,67.6 41.7,67.5 R204.2 41.2,67.5 41,67.7 41,69.43 40.68,69.75 39.95,69.75 39.8,69.6 D202-.2 D203-.5 39.8,65.4 39.79,65.4 39.64,65.25 38.75,65.25 38.4,65.6 38.4,67 37.9,67.5 C203.2 36.65,66.65 36.3,66.3 34.1,66.3 33.5,65.7 33.5,61.7 32.7,60.9 22.2,60.9 21.4,60.1 v21.4,49.5 | INTERFACE_TO_UC/MC.17 2.89,37.09 3.2,37.4 v12.4,37.4
  Bottom 0.3: v12.4,48 v12.4,37.4 | v21.4,48 v21.4,49.5
GND  (via drill 0.3 pad 0.3, 3.2 pad 6.35)
  Top 0.3: IC3.6 25.15,42.75 25.2,42.7 27.3,42.7 IC3.49 | IC3.18 27.25,42.25 IC3.49 | IC3.43 27.25,42.75 IC3.49 | IC3.34 29.25,44.25 IC3.49 | IC3.24 30.25,39.75 IC3.49 | D203-.1 39.73,64.15 D203-.2 40.27,64.08 D203-.3 | D305-.1 39.34,14.08 D305-.2 40.28,14.08 40.3,14.1 40.4,14.1 | v26.5,43.5 26.5,42.75 IC3.31 33.47,42.75 35.02,41.2 35.3,41.2 35.75,41.65 C311.1 | IC3.48 24.75,45.25 v25.5,44.5 | IC3.38 29.75,44.75 v29.5,44.5 | IC3.13 24.75,39.75 v25.5,40.5
  other vias: 26.5,44.5 25.5,42.5 25.5,43.5 26.5,40.5 27.5,40.5 29.5,40.5 25.5,41.5 28.5,40.5 29.5,43.5 28.5,44.5 27.5,44.5 29.5,42.5 29.5,41.5 27.5,41.5 26.5,42.5 27.5,42.5 28.5,42.5 27.5,43.5 23.75,54 24.75,54 25.75,54 28.75,54 29.75,54 30.75,54 23.75,31 24.75,31 25.75,31 29.75,31 30.75,31 28.75,31 40,57.5 26.5,41.5 28.5,41.5 28.5,43.5 27.15,32.2 26.75,52.3 4,4 51,4 51,81 4,81 30,82.5 35,82.5 40,82.5 45,82.5 45,77.5 40,77.5 35,77.5 31.9,77.5 25.8,77.5 20,82.5 2.5,77.5 2.5,72.5 33.6,26.7 45,60 40,62.5 40,40 52.5,57.5 35,58.5 25,58.5 12.19,57.5 52.5,52.5 52.5,47.5 52.5,42.5 40,47.5 52.5,37.5 42.5,37.3 40,37.3 15,37.5 15,32.5 52.5,32.5 52.5,27.5 42.5,32.5 24.5,26.2 30,17.5 17.5,17.5 12.5,17.5 30,12.5 37.5,12.5 47.5,12.5 45,7.5 37.5,7.5 30,7.5 15,2.5 2.5,7.5 37.5,2.5 47.5,2.5 30,2.5 22.5,2.5 12.5,22.5 40,51.25 30,67.5 35,62.5 17.85,45.95 30,70 30,58.5 20.3,70 16.6,66.6 23.2,59.1 20.3,61.7 20,58.5 34.9,53.7 17.5,20 12.5,20 25,17.5 17.5,29.3 17.5,10 22.5,15 41.4,25 42.5,27.5 47.5,32.5 5,12.5 10,12.5 12.5,7.5 25,82.5 10,82.5 17.5,77.5 25.8,70 10,77.5 20.3,72.5 12.19,64.06 10,72.5 17.5,72.5 17.5,70 14.16,66.6 25,67.5 15,82.5 13.75,43.75 12.19,50 17.64,50 42.5,12.5 47.5,37.5 34.7,73.1 45,66.25 45,68.75 45,71.25 44.99,21.1 45.01,18.79 44.97,16.32 22.73,10.01 2.8,19.68 29.2,73 25.8,72.5 47.5,27.5 14.06,57.5 14.06,50 30,25 23.4,25.1 17.5,25 23.1,72.5 23.1,70 16.6,61.7 20.3,66.6
  pour Top: 0,85 55,85 55,0 0,0
  pour Bottom: 0.2,85 55,85 55,0 0,0
  pour Route2: 0,85 55,85 55,0 0,0
ID_CH0  (via drill 0.3 pad 0.3)
  Top 0.3: 8.61,20.9 8.9,20.9 v18.7,20.9 | IC1.5 21.93,6 v23.9,6
  Top 0.5: INTERFACE_TO_UC/MC.6 8.9,20.9
  Bottom 0.3: v23.9,6 23.9,15.7 v18.7,20.9
ID_CLK  (via drill 0.3)
  Top 0.3: R211.1 16.3,7.9 v16.6,7.6 16.88,7.33 IC1.2 | INTERFACE_TO_UC/MC.4 13.93,18.37 v16.6,15.7
  Bottom 0.3: v16.6,7.6 v16.6,15.7
N$1
  Top 0.3: C207.1 14.2,8.6 16.12,6.67 IC1.3 19.38,6.67 19.9,7.2 R212.2
N$2
  Top 0.3: R213.1 24.5,8 23.82,7.33 | IC1.7 23.82,7.33 | C208.1 26.6,8.1 25.82,7.33 23.82,7.33
N$3  (via drill 0.3 pad 0.3)
  Top 0.3: R203.1 v45.3,70 R207.1
  Bottom 0.3: v45.3,70 47.92,70 ENCODER1.5
N$4  (via drill 0.3 pad 0.3)
  Top 0.3: R204.1 v45.3,67.5 R208.1
  Bottom 0.3: v45.3,67.5 47.96,67.5 ENCODER1.4
N$5  (via drill 0.3 pad 0.3)
  Top 0.3: R205.1 v45.3,65 R209.1
  Bottom 0.3: v45.3,65 48,65 ENCODER1.3
N$6  (via drill 0.3 pad 0.3)
  Top 0.3: R206.1 v45.3,20 R210.1
  Bottom 0.3: v45.3,20 50.92,20 ENCODER2.5
N$7  (via drill 0.3 pad 0.3)
  Top 0.3: R222.1 v45.3,17.5 R219.1
  Bottom 0.3: v45.3,17.5 50.96,17.5 ENCODER2.4
N$8  (via drill 0.3 pad 0.3)
  Top 0.3: R223.1 v45.3,15 R220.1
  Bottom 0.3: v45.3,15 51,15 ENCODER2.3
N$9
  Top 0.3: 38.4,42.5 36.2,40.3
O1A1  (via drill 0.3 pad 0.3)
  Top 0.3: IC3.47 25.25,46.62 23.92,47.95 v23.8,47.95
  Top 0.7: v24.5,47.1 23.8,47.8 v23.8,47.95
  Bottom 0.7: v23.8,47.95 23.8,47.8 v24.5,47.1 26.15,45.45 44.4,45.45 MOTOR1.1
O1A2  (via drill 0.3 pad 0.3)
  Top 0.3: IC3.45 v26.25,47.45
  Top 0.7: v26.25,47.45 v26.25,48.45
  Bottom 0.7: MOTOR1.2 36,50.25 32.1,46.35 26.65,46.35 26.25,46.75 v26.25,47.45 v26.25,48.45
O1B1  (via drill 0.3 pad 0.3)
  Top 0.3: IC3.41 v28.25,47.45
  Top 0.7: v28.25,47.45 v28.25,48.45
  Bottom 0.7: MOTOR1.3 44.45,52.5 36.55,52.5 31.3,47.25 28.45,47.25 v28.25,47.45 v28.25,48.45 28.25,48.25 29.1,47.4
O1B2  (via drill 0.3 pad 0.3)
  Top 0.3: IC3.39 29.25,46.7 v31.6,49.05
  Top 0.7: v30.9,48.2 31.6,48.9 31.6,49
  Bottom 0.7: MOTOR1.4 42.15,53.7 36.25,53.7 v31.6,49.05 31.6,48.9 v30.9,48.2
O2A1  (via drill 0.3 pad 0.3)
  Top 0.3: IC3.14 25.25,38.45 23.95,37.15 v23.8,37.15
  Top 0.7: v24.5,37.9 23.8,37.2 v23.8,37.15
  Bottom 0.7: MOTOR2.1 40.95,32.5 28.45,32.5 24.57,36.38 24.5,36.45 | 24.5,36.45 v23.8,37.15 | 23.8,37.2 v24.5,37.9 24.5,36.45
O2A2  (via drill 0.3 pad 0.3)
  Top 0.3: IC3.16 v26.25,37.45
  Top 0.7: v26.25,37.45 v26.25,36.45
  Bottom 0.7: v26.25,37.45 v26.25,36.45 29,33.7 43.25,33.7 MOTOR2.2
O2B1  (via drill 0.3 pad 0.3)
  Top 0.3: IC3.20 v28.25,37.45
  Top 0.7: v28.25,37.45 v28.25,36.45
  Bottom 0.7: 28.25,36.6 v28.25,36.45 | v28.25,36.45 v28.25,37.45 | v28.25,36.45 29.9,34.8 45.65,34.8 MOTOR2.3
O2B2  (via drill 0.3 pad 0.3)
  Top 0.3: IC3.22 29.25,38.35 30.45,37.15 v30.7,37.15
  Top 0.7: v30,37.9 30.7,37.2 v30.7,37.15
  Bottom 0.7: MOTOR2.4 43.35,35.9 31.95,35.9 v30.7,37.15 30.7,37.2 v30,37.9 30,37.83
REFL1/STEP1  (via drill 0.3 pad 0.25, 0.3 pad 0.3)
  Top 0.3: D203-.6 D202-.1 39.3,69.19 39.3,69.7 39.15,69.85 | C202.2 v37.9,70 39,70 39.15,69.85 | IC3.28 32.05,41.25 32.8,40.5 32.8,38.74 v33.34,38.2 | 39.15,69.85 39.55,70.25 40.95,70.25 41.2,70 R203.2
  Bottom 0.3: v33.34,38.2 42.6,38.2 47.5,43.1 47.5,60.4 45.2,62.7 41.2,62.7 37.9,66 v37.9,70
REFL2/STEP2  (via drill 0.3 pad 0.25)
  Top 0.3: D305-.6 D204-.1 39.26,19.69 39.02,19.93 | 39.02,19.93 38.95,20 v37.9,20 C205.2 | 41.9,20 R206.2 41.7,20.25 39.55,20.25 39.23,19.93 39.02,19.93 | IC3.26 31.57,40.25 31.75,40.07 31.75,37.95 33.6,36.1 33.6,31.9 37.83,27.67 arc-45 37.9,27.5 v37.9,25.5
  Bottom 0.3: v37.9,20 v37.9,25.5
REFR1/DIR1  (via drill 0.3 pad 0.25, 0.3 pad 0.3)
  Top 0.3: D305-.4 D204-.3 | D305-.4 | R223.2 40.63,15 40.47,15.16 | 40.47,15.16 40.35,15.28 40.35,15.84 D305-.4 | 36.9,14.75 arc-90 C221.2 36.9,14.75 | IC3.27 31.85,40.75 32.3,40.3 32.3,38.2 35.2,35.3 v35.2,31.45 | 36.9,14.75 v37.9,14.75 40.05,14.75 40.47,15.16
  Bottom 0.3: v37.9,14.75 35.2,17.45 v35.2,31.45
REFR2/DIR2  (via drill 0.3 pad 0.25, 0.3 pad 0.3)
  Top 0.3: D305-.5 D204-.2 39.8,19.61 39.94,19.75 40.69,19.75 41,19.44 41,19.2 41.95,18.25 R222.2 | 39.8,15.5 D305-.5 | 39.8,15.47 D305-.5 | D305-.5 39.8,15.41 39.64,15.25 38.8,15.25 38.32,15.73 38.32,17.08 v37.9,17.5 C220.2 | IC3.25 31,37.9 32,36.9 32,32.4 36.98,27.42 arc-45 37.05,27.25 v37.05,26.15
  Bottom 0.3: v37.9,17.5 37.55,17.85 37.12,18.28 | 37.12,18.28 37.1,18.3 | v37.05,26.15 37.05,18.45 arc45 37.12,18.28
SPI1_CSN  (via drill 0.3 pad 0.3)
  Top 0.3: INTERFACE_TO_UC/MC.30 19.91,51.39 v20.3,51 | IC3.3 22.78,44.25 20.3,46.73 v20.3,47.25
  Bottom 0.3: v20.3,47.25 v20.3,51
SPI1_SCK  (via drill 0.3 pad 0.3)
  Top 0.3: INTERFACE_TO_UC/MC.31 2.89,53.01 3.2,52.7 18.8,52.7 v19.2,52.3 | IC3.4 22.5,43.75 22.5,43.8 v19.2,47.1
  Bottom 0.3: v19.2,47.1 v19.2,52.3
SPI1_SDI  (via drill 0.3 pad 0.25)
  Top 0.3: IC3.5 21.95,43.25 v19.7,45.5 | v18.4,53.43 17.9,53.93 INTERFACE_TO_UC/MC.32
  Bottom 0.3: v18.4,53.43 18.4,46.8 v19.7,45.5
SPI1_SDO  (via drill 0.3 pad 0.3)
  Top 0.3: INTERFACE_TO_UC/MC.33 2.89,55.61 3.2,55.3 v16.9,55.3 | IC3.8 19.95,41.75 v16.9,44.8
  Bottom 0.3: v16.9,44.8 v16.9,55.3
SWION  (via drill 0.3, 0.3 pad 0.3)
  Top 0.3: INTERFACE_TO_UC/MC.41 2.89,65.51 3.1,65.3 v13.19,65.3 13.19,78.15 CON_SW.3 | IC3.10 18.4,40.75 13.19,45.96 v13.19,46.5
  Bottom 0.3: v13.19,46.5 v13.19,65.3
SWIOP  (via drill 0.3, 0.3 pad 0.3)
  Top 0.3: INTERFACE_TO_UC/MC.40 9.1,62.8 | INTERFACE_TO_UC/MC.39 2.89,63.11 3.2,62.8 9.1,62.8 | IC3.9 19.26,41.25 15.01,45.5 v15.01,46.5 | 9.1,62.8 v15.01,62.8 15.01,77.51 CON_SW.1
  Bottom 0.3: v15.01,46.5 v15.01,62.8
SWSEL  (via drill 0.3 pad 0.3)
  Top 0.3: IC3.12 16.8,39.75 v15.8,40.74 | D202-1.5 14.9,61.48 v15.8,60.58 | v15.8,60.58 15.8,71.6 15.8,73.22 15.8,73.28 SW_SEL.2 | R321.2 14.84,59.61 v15.8,60.58
  Bottom 0.3: v15.8,40.74 v15.8,60.58
VCC
  Top 0.3: IC3.33 33.28,43.75 33.84,44.31 C310.2 arc90 34.1,44.1 35.7,44.1 arc-90 35.85,44.25 R311.1
VCC_IO  (via drill 0.3 pad 0.3)
  Top 0.3: IC3.7 23.35,42.25 23,42.6 | 39.8,72.1 39.77,72.1 | D202-.6 39.26,70.99
  Top 0.5: D202-.5 40.26,70.92 D202-.4 | D202-.5 39.34,70.92 D202-.6 | R220.2 R219.2 R210.2 48.7,20.05 48.7,22 | 48.7,22 39.8,22 | 39.8,22 D204-.5 | D204-.5 40.26,20.93 D204-.4 | D204-.5 39.34,20.93 D204-.6 | 39.8,22 v21.27,22 v21.27,16.09 19.06,16.09 18.35,15.38 R202.1 | 23,42.6 v21.27,42.6 20.5,42.6 C101.2 | D202-.5 39.8,72.1 47.6,72.1 48.65,71.05 R207.2 R208.2 R209.2 48.7,64.95 48.7,22 | 39.77,72.1 28.5,72.1 24.57,76.03 SW_SEL.1
  Bottom 0.3: v21.27,16.09 21.27,4.11 TEST_POINT5.P$1
  Bottom 0.5: v21.27,42.6 v21.27,22
VCP
  Top 0.3: IC3.37 31,46 31.8,46.8 31.8,48 32.2,48.4 32.4,48.4 32.81,48.81 C307.1
VM  (via drill 0.3 pad 0.3)
  Top 0.3: C308.2 v27.25,37.79 v27.24,37.8 | IC3.17 26.75,38.29 v27.24,37.8 | IC3.19 27.75,38.31 v27.24,37.8 | INTERFACE_TO_UC/MC.1 v2.89,13.28 | IC3.30 32.95,42.25 v33.2,42 v33.9,41.3 34.9,40.3 C312.2 | v36.62,48.17 v36.62,49.17 34.67,49.17 34.52,49.32 C307.2 | IC3.44 26.75,46.81 v27.24,47.3 | IC3.42 27.75,46.79 v27.24,47.3 | v27.24,47.3 v27.24,48.29 v27.25,48.3 C309.2
  Top 0.5: v33,73.88 v33,73.89 v32,73.89 | v32,73.88 v32,73.89 | v32,73.89 v30.99,73.89 30.99,73.9 30,73.9 | v31,73.88 31,75 D1.C 32,75 32,73.9
  other vias: 27.24,36.8 30,73.88
  pour Route3 (isolate 0.1): 0,85 55,85 55,0 0,0

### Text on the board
tPlace: 7..18V | GND | L1 | N | +VM | GND | B | A | GND | ENC1 | +5V | B2 | B1 | A2 | A1 | GND | B2 | GND | B1 | A2 | A1 | L2 | N | R2 | B | R1 | A | GND | GND | ENC2 | +5V | TMC5062-Eval v1.3
bPlace: TMC-Evaluation-Platform: | TMC5062-Eval | Interfaces: | SPI, SW-UART | Voltage: | 7V...18V | Current: | 2x1.1A RMS | v1.2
